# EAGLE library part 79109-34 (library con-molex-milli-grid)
RECEPTACAL
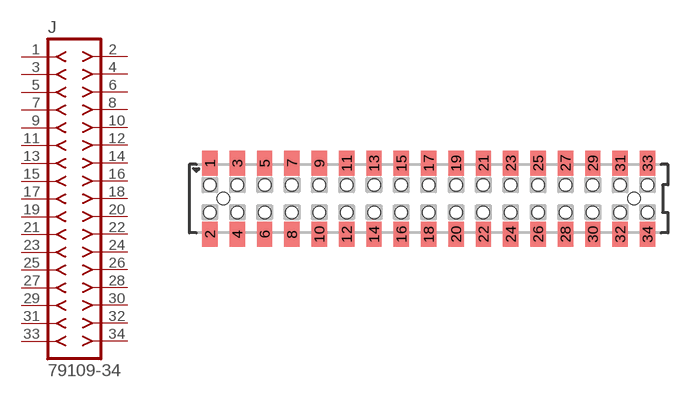
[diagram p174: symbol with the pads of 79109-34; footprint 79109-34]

Designator prefix J

## 79109-34  [79109-34]
1  1  pas
2  2  pas
3  3  pas
4  4  pas
5  5  pas
6  6  pas
7  7  pas
8  8  pas
9  9  pas
10  10  pas
11  11  pas
12  12  pas
13  13  pas
14  14  pas
15  15  pas
16  16  pas
17  17  pas
18  18  pas
19  19  pas
20  20  pas
21  21  pas
22  22  pas
23  23  pas
24  24  pas
25  25  pas
26  26  pas
27  27  pas
28  28  pas
29  29  pas
30  30  pas
31  31  pas
32  32  pas
33  33  pas
34  34  pas

## Footprint 79109-34 (pad centres in mm)
RECEPTACAL SMD Dual Row, Vertical, Pass-Thru
smd 1.12 x 1.83: 1 -16,2.6; 2 -16,-2.6; 3 -14,2.6; 4 -14,-2.6; 5 -12,2.6; 6 -12,-2.6; 7 -10,2.6; 8 -10,-2.6; 9 -8,2.6; 10 -8,-2.6; 11 -6,2.6; 12 -6,-2.6; 13 -4,2.6; 14 -4,-2.6; 15 -2,2.6; 16 -2,-2.6; 17 0,2.6; 18 0,-2.6; 19 2,2.6; 20 2,-2.6; 21 4,2.6; 22 4,-2.6; 23 6,2.6; 24 6,-2.6; 25 8,2.6; 26 8,-2.6; 27 10,2.6; 28 10,-2.6; 29 12,2.6; 30 12,-2.6; 31 14,2.6; 32 14,-2.6; 33 16,2.6; 34 16,-2.6
hole 0.914 at -15,0
hole 0.914 at -16,1
hole 0.914 at -16,-1
hole 0.914 at -14,-1
hole 0.914 at -14,1
hole 0.914 at -12,-1
hole 0.914 at -12,1
hole 0.914 at 15,0
hole 0.914 at -10,1
hole 0.914 at -10,-1
hole 0.914 at -8,1
hole 0.914 at -8,-1
hole 0.914 at -6,1
hole 0.914 at -6,-1
hole 0.914 at -4,1
hole 0.914 at -4,-1
hole 0.914 at -2,-1
hole 0.914 at -2,1
hole 0.914 at 0,1
hole 0.914 at 0,-1
hole 0.914 at 2,1
hole 0.914 at 2,-1
hole 0.914 at 4,1
hole 0.914 at 4,-1
hole 0.914 at 6,-1
hole 0.914 at 6,1
hole 0.914 at 8,1
hole 0.914 at 10,1
hole 0.914 at 12,1
hole 0.914 at 8,-1
hole 0.914 at 10,-1
hole 0.914 at 12,-1
hole 0.914 at 14,-1
hole 0.914 at 16,-1
hole 0.914 at 14,1
hole 0.914 at 16,1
